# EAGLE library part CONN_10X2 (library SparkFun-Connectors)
Multi connection point. Often used as Generic Header-pin footprint for 0.1 inch spaced/style header connections On any of the 0.1 inch spaced packages, you can populate with these: Break Away Headers - Straight (PRT-00116) Break Away Male Headers - Right Angle (PRT-00553) Female Headers (PRT-00115) Break Away Headers - Machine Pin (PRT-00117) Break Away Female Headers - Swiss Machine Pin (PRT-00743) Special note about the "SPECIAL" package: This was SPECIALLY designed to be used with our Graphic LCD Backpack. Be sure you want to use this! It is not only staggered on each line of header holes, but IT IS ALSO offset of the center point of the top and bottom lines by 5 mil. This causes the headers to lock into place on the "standard" footprint on the LCD screen. The extra squares on the tdocu layer are there simply to reference other pins (if you were to actually populate a longer header than ten long - this is what we do with the backpacks).
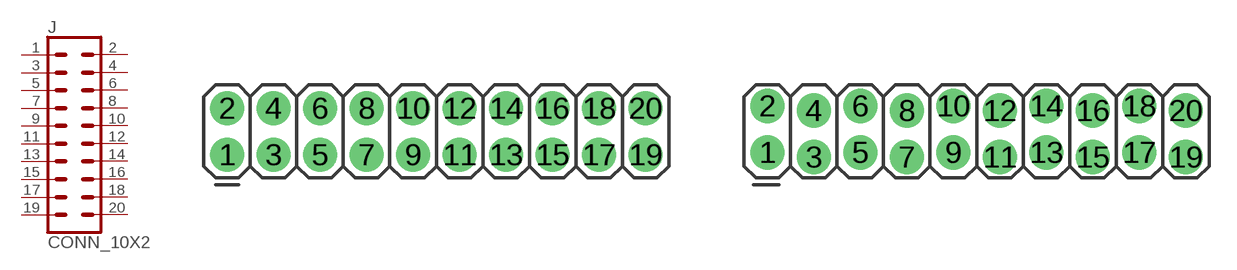
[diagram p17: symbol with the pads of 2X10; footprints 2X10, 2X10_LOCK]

Designator prefix J

## CONN_10X2  [2X10]
1  1  pas
2  2  pas
3  3  pas
4  4  pas
5  5  pas
6  6  pas
7  7  pas
8  8  pas
9  9  pas
10  10  pas
11  11  pas
12  12  pas
13  13  pas
14  14  pas
15  15  pas
16  16  pas
17  17  pas
18  18  pas
19  19  pas
20  20  pas

## CONN_10X22X10_LOCK  [2X10_LOCK]
Pads as for 2X10

## CONN_10X2SPECIAL  [2X10_LOCK_SPECIAL]
Pads as for 2X10

## CONN_10X2NOSILK  [2X10_NOSILK]
Pads as for 2X10

## Footprint 2X10 (pad centres in mm)
Plated Through Hole - 2x10 Specifications: Pin count:20 Pin pitch:0.1" Example device(s): CONN_10x2
drill 1.016 pad 1.88: 1 0,0; 2 0,2.54; 3 2.54,0; 4 2.54,2.54; 5 5.08,0; 6 5.08,2.54; 7 7.62,0; 8 7.62,2.54; 9 10.16,0; 10 10.16,2.54; 11 12.7,0; 12 12.7,2.54; 13 15.24,0; 14 15.24,2.54; 15 17.78,0; 16 17.78,2.54; 17 20.32,0; 18 20.32,2.54; 19 22.86,0; 20 22.86,2.54

## Footprint 2X10_LOCK (pad centres in mm)
Plated Through Hole - 2x10 Locking Footprint Holes are offset 0.005", to hold pins in place while soldering. Specifications: Pin count:20 Pin pitch:0.1" Example device(s): CONN_10x2
drill 1.016 pad 1.88: 1 0,0.127; 2 0,2.667; 3 2.54,-0.127; 4 2.54,2.413; 5 5.08,0.127; 6 5.08,2.667; 7 7.62,-0.127; 8 7.62,2.413; 9 10.16,0.127; 10 10.16,2.667; 11 12.7,-0.127; 12 12.7,2.413; 13 15.24,0.127; 14 15.24,2.667; 15 17.78,-0.127; 16 17.78,2.413; 17 20.32,0.127; 18 20.32,2.667; 19 22.86,-0.127; 20 22.86,2.413

## Footprint 2X10_LOCK_SPECIAL (pad centres in mm)
Plated Through Hole - 2x10 Locking Footprint Special Holes are offset 0.005", to hold pins in place while soldering. Pin rows are offset 5mm as well Specifications: Pin count:20 Pin pitch:0.1"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
drill 1.016 pad 1.88: 1 0,-0.152; 2 0,2.946; 3 2.54,-0.406; 4 2.54,2.692; 5 5.08,-0.152; 6 5.08,2.946; 7 7.62,-0.406; 8 7.62,2.692; 9 10.16,-0.152; 10 10.16,2.946; 11 12.7,-0.406; 12 12.7,2.692; 13 15.24,-0.152; 14 15.24,2.946; 15 17.78,-0.406; 16 17.78,2.692; 17 20.32,-0.152; 18 20.32,2.946; 19 22.86,-0.406; 20 22.86,2.692

## Footprint 2X10_NOSILK (pad centres in mm)
Plated Through Hole - 2x10 No Silk Outline Specifications: Pin count:20 Pin pitch:0.1" Example device(s): CONN_10x2
drill 1.016 pad 1.88: 1 0,0; 2 0,2.54; 3 2.54,0; 4 2.54,2.54; 5 5.08,0; 6 5.08,2.54; 7 7.62,0; 8 7.62,2.54; 9 10.16,0; 10 10.16,2.54; 11 12.7,0; 12 12.7,2.54; 13 15.24,0; 14 15.24,2.54; 15 17.78,0; 16 17.78,2.54; 17 20.32,0; 18 20.32,2.54; 19 22.86,0; 20 22.86,2.54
